(* Logix 5000 AddOnInstructionDefinition export EGU_EGK_Cyclic_Communication_1_0_3; software revision 35.00 *)

ADD_ON_INSTRUCTION EGU_EGK_Cyclic_Communication_1_0_3   (* revision 1.0 3, ExecutePrescan, ExecuteEnableInFalse *)
// Release 5.3.xxx
// ussed for EG Tested with:   V29.00.01 (CPR 9 SR 8.1) Built on: 08/11/16 01:38:38
//                 Schunk FW release 5.x
//  Engineering:   Studio 5000 V29.00.01 (CPR 9 SR 8.1) Built on: 08/11/16 01:38:38U / EGK Gripper
// Revision note:
// Change for Firmware 5.3
VAR_INPUT
   b_in_RELEASE_FUNCTION_BLOCK : BOOL; {access Read Only, visible}
   b_in_00_FAST_STOP : BOOL; {access Read Only, visible}
   b_in_01_STOP : BOOL; {access Read Only, visible}
   b_in_02_ACKNOLEDGE : BOOL; {access Read Only, visible}
   b_in_03_PREPARE_FOR_SHUTDOWN : BOOL; {access Read Only, visible}
   b_in_04_SOFTRESET : BOOL; {access Read Only, visible}
   b_in_05_RELEASE_FOR_MANUAL_MOVEMENT : BOOL; {access Read Only, visible}
   b_in_06_REPEAT_COMMAND_TOGGLE : BOOL; {access Read Only, visible}
   b_in_07_GRIP_DIRECTION : BOOL; {access Read Only, visible}
   b_in_08_JOG_MODE_NEGATIVE : BOOL; {access Read Only, visible}
   b_in_09_JOG_MODE_POSITIVE : BOOL; {access Read Only, visible}
   b_in_11_RELEASE_WORKPIECE : BOOL; {access Read Only, visible}
   b_in_12_GRIP_WORKPIECE : BOOL; {access Read Only, visible}
   b_in_13_MOVE_TO_ABSOLUTE_POSITION : BOOL; {access Read Only, visible}
   b_in_14_MOVE_TO_RELATIVE_POSITION : BOOL; {access Read Only, visible}
   b_in_16_GRIP_WORKPIECE_AT_EXPECTED_POS : BOOL; {access Read Only, visible}
   b_in_30_BRAKE_TEST : BOOL; {access Read Only, visible}
   b_in_31_ACTIVATE_GRIP_FORCE_AND_POS_MA : BOOL; {access Read Only, visible}
   di_in_POSITION : DINT; {access Read Only, visible}
   di_in_VELOCITY : DINT; {access Read Only, visible}
   di_in_GRIPPING_FORCE : DINT; {access Read Only, visible}
END_VAR
VAR_OUTPUT
   b_out_00_READY_FOR_OPERATION : BOOL; {visible}
   b_out_01_CONTOL_AUTHORITY_FIELDBUS : BOOL; {visible}
   b_out_02_READY_FOR_SHUTDOWN : BOOL; {visible}
   b_out_03_NOT_FEASIBLE : BOOL; {visible}
   b_out_04_COMMAND_SUCCESSFULLY_PROCESSED : BOOL; {visible}
   b_out_05_COMMAND_RECEIVED_TOGGLE : BOOL; {visible}
   b_out_06_WARNING : BOOL; {visible}
   b_out_07_ERROR : BOOL; {visible}
   b_out_08_RELEASED_FOR_MANUAL_MOVEMENT : BOOL; {visible}
   b_out_09_SOFTWARE_LIMIT_REACHED : BOOL; {visible}
   b_out_11_NO_WORKPIECE_DETECTED : BOOL; {visible}
   b_out_12_WORKPIECE_GRIPPED : BOOL; {visible}
   b_out_13_POSITION_REACHED : BOOL; {visible}
   b_out_14_WORKPIECE_PRE_GRIP_STARTED : BOOL; {visible}
   b_out_16_WORKPIECE_LOST : BOOL; {visible}
   b_out_17_WRONG_WORKPIECE_DETECTED : BOOL; {visible}
   b_out_31_GRIP_FORCE_AND_POS_MAINTAINANC : BOOL; {visible}
END_VAR
VAR_INPUT
   di_out_ACTUAL_POSITION : DINT; {visible}
END_VAR
VAR_OUTPUT
   si_out_DIAGNOSIS_ERROR : SINT; {visible}
   si_out_DIAGNOSIS_WARNING : SINT; {visible}
   si_out_DIAGNOSIS_WARNING_CODE : SINT; {visible}
END_VAR
VAR_INPUT
   di_in_INPUT_DATA_GRIPPER_DW_0 : DINT; {access Read Only, required}
   di_in_INPUT_DATA_GRIPPER_DW_1 : DINT; {access Read Only, required}
   di_in_INPUT_DATA_GRIPPER_DW_3 : DINT; {access Read Only, required}
END_VAR
VAR_OUTPUT
   di_out_OUTPUT_DATA_Gripper_DW_0 : DINT; {required}
   di_out_OUTPUT_DATA_Gripper_DW_1 : DINT; {required}
   di_out_OUTPUT_DATA_Gripper_DW_2 : DINT; {required}
   di_out_OUTPUT_DATA_Gripper_DW_3 : DINT; {required}
END_VAR
VAR
   stat_Input : DINT[4]; {access None}
   stat_Output : DINT[4]; {access None}
END_VAR

ROUTINE EnableInFalse   (* structured text *)
   //////////////////////////////////////////////////////////////
   //   Copyright (c)  <Company Information>
   //--------------------------------------------------------------
   //   Routine: <Routine Name>
   //       Author: <Developer Name>
   //   Created: <Date>
   //--------------------------------------------------------------
   //   Description:
   //
   //   History:
   //
   /////////////////////////////////////////////////////////////
END_ROUTINE

ROUTINE Logic   (* structured text *)
   
   (*
   FUNCTION_BLOCK FB_SFP_EGU/EGK Allen Breadley
   TITLE = 'EGU_EGK_Cyclic_Communication'
   VERSION : '1.0.3'
   AUTHOR  : 'SCHUNK'
   NAME    : 'EGU_EGK_Cyclic_Communication'
   FAMILY  : 'SCHUNK'
   Used Products : EGU / EGK
   Projekt Nr.:
   =============================================================================
    Schunk GmbH&Co.KG
    (c)Copyright (2022) All Rights Reserved
   -----------------------------------------------------------------------------
    Library:       Schunk
    Tested with:   V35.00.00
                   Schunk FW release 5.x
    Engineering:   Studio 5000 V35.00.00
    Restrictions:  XXX(OB types, etc.)
    Requirements:  (hardware, technological package, memory needed, etc.)
    Functionality: The Funktion Block communicates Cyclic with the Gripper to read and wright Data
   
   *************************************************************************
   Historie
   ####################
   1.0.3
   - Compartible with FW 5.3 Protokol
   - order when deleting bits changed
   ####################
   1.0.2
   - Compartible with FW 5.2 Protokol
   - New Bit "Brake Test"
   - Changesd Bit Names not the Funktions behind
   ####################
   1.0.1
   Bugfix
   	di_out_OUTPUT_DATA_Gripper_DW_2 := di_in_VELOCITY;
   	di_out_OUTPUT_DATA_Gripper_DW_3 := di_in_GRIPPING_FORCE;
   ####################
   1.0.0
   Release Funktion Block
   TagType="Base" DataType="BOOL" Usage="Input" Radix="Binary" Required="false" Visible="true" ExternalAccess="Read Only"
   
   *************************************************************************)
   	(*English
   
       Statement section REGION
   
       *************************************************************************
       The function block is TO read AND transfer cyclic parameters that are changed FOR specific functions in the device
       can be used TO make The application process safer OR faster.
   
       Input parameters:
       ------------------
       b_in_RELEASE_FUNCTION_BLOCK				: Release FOR processing the block
   
       b_in_00_FAST_STOP						: immediate shutdown OF The process currently running in The gripper AND shutdown OF The motor phases
       b_in_01_STOP							: Pausing AND stopping the currently running process.
       b_in_02_ACKNOLEDGE						: Acknowledge fault
       b_in_03_PREPARE_FOR_SHUTDOWN			: Initiate the restoration OF data on The device in preparation FOR switching off OR rebooting
       b_in_04_SOFTRESET						: Warm start OF The device
       b_in_05_RELEASE_FOR_MANUAL_MOVEMENT		: The brake can be released FOR 5 seconds in the "ERROR_FAST_STOP" state
       b_in_06_REPEAT_COMMAND_TOGGLE			: The command that is still pending can, IF it is a repeatable command, be repeated without loss OF Time FOR each positive AND negative change OF this bit
       b_in_07_GRIP_DIRECTION					: determines The gripping direction. FALSE = external gripping (the workpiece is gripped from the outside) / True = internal gripping (the workpiece is gripped from the inside).
   
       b_in_08_JOG_MODE_NEGATIVE				: Simple movement OF The device in negative direction. Function also possible without "REFERENCE".
       b_in_09_JOG_MODE_POSITIVE				: Simple movement OF The device in The positive direction. Function also possible without "REFERENCE".
   
       b_in_11_RELEASE_WORKPIECE				: IF The status is "GRIPPED", the gripper is opened in the opposite direction AND the workpiece is released
       b_in_12_GRIP_WORKPIECE					: the gripper executes a movement that should lead TO gripping a workpiece. Internal speed parameters are used here
       b_in_13_MOVE_TO_ABSOLUTE_POSITION		: the gripper jaws are moved TO The position specified in The cyclic protocol at The specified speed.
       b_in_14_MOVE_TO_RELATIVE_POSITION		: the gripper jaws are moved TO The calculated position with The position specified in The cyclic protocol at The specified speed.
   
       b_in_16_GRIP_WORKPIECE_AT_EXPECTED_POSITION :  the gripper performs a gripping run on a specified workpiece. first a positioning run to the pre-position and then a gripping run to the workpiece.
       b_in_30_BRAKE_TEST						: the gripper activates the brake and energizes the motor
   	b_in_31_ACTIVATE_GRIP_FORCE_AND_POSITION_MAINTENANCE  :  sets the use of gripping force and position maintenance ( False = GPE is not used / True = GPE is activated)
   
       di_in_POSITION							: Entry of the absolute or relative position in µm
       di_in_VELOCITY							: Entry of the speed when positioning gripping mm/sec
       di_in_GRIPPING_FORCE					: Entry of the gripping force is entered in %. Here you can read in the manual which gripping modes should be used. The indication of the gripping force can then be selected accordingly.
   
       di_in_INPUT_DATA_GRIPPER_DW_0			: Input Data DoubleWord 0 of the Gripper
       di_in_INPUT_DATA_GRIPPER_DW_1			: Input Data DoubleWord 1 of the Gripper
       di_in_INPUT_DATA_GRIPPER_DW_2			: Input Data DoubleWord 2 of the Gripper
       di_in_INPUT_DATA_GRIPPER_DW_3			: Input Data DoubleWord 3 of the Gripper
   
       #################
   
       Output parameters:
       ------------------
   
       b_out_00_READY_FOR_OPERATION            : indicates that the gripper is ready FOR operation
       b_out_01_CONTOL_AUTHORITY_FIELDBUS      : indicates whether the fieldbus has control authority over the gripper
       b_out_02_READY_FOR_SHUTDOWN             : signals readiness FOR shutdown OR restart after the request "Prepare for shutdown"
       b_out_03_NOT_FEASIBLE                   : Indicates that the last issued command cannot be executed.
                                               Possible causes are:
                                               - a new command was sent although the command that is still active has NOT yet been processed.
                                               - 2 OR more control commands simultaneously active in the control word
                                               - Parameter data FOR position, speed OR force are outside the permissible limits.
   
       b_out_04_COMMAND_SUCCESSFULLY_PROCESSED : indicates that the last executable command was successfully processed.
       b_out_05_COMMAND_RECEIVED_TOGGLE        : indicates that a command was sent TO The gripper via The bus. the command does NOT have TO be processed OR started at the time it is displayed.
       b_out_06_WARNING                        : signals a warning in the gripper, e.g. temperature warning
       b_out_07_ERROR                          : signals a fault in the gripper, e.g. rapid stop
       b_out_08_RELEASD_FOR_MANUAL_MOVEMENT    : Signals that the brake is released IF a brake is installed in the gripper.
       b_out_09_SOFTWARELIMIT_REACHED          : indicates that the gripper has reached a software limit
   
       b_out_11_NO_WORKPIECE_DETECTED          : indicates that no workpiece was detected
       b_out_12_WORKPIECE_GRIPPED              : signals that a workpiece has been gripped
       b_out_13_POSITION_REACHED               : signals that the relative OR absolute position has been approached
       b_out_14_WORKPIECE_PRE_GRIPPED_STARTED  : indicates that the gripper has started the pre-gripping function
       b_out_16_WORKPIECE_LOST                 : signals that the gripped workpiece was lost
       b_out_17_WRONG_WORKPIECE_DETECTED       : signals that a wrong workpiece was detected
       b_out_31_GRIP_FORCE_AND_POSITION_MAINTAINANCE_ACTIVATED : signals that GPE is active
   
       di_out_ACTUAL_POSITION                  : the current position OF The gripper is returned here
       i_out_DIAGNOSE_WARNUNG                  : Output of the gripper's warning code
       i_out_DIAGNOSE_ERROR                    : Output of the error code of the gripper
   
       di_out_OUTPUT_DATA_Gripper_DW_0			: Output Data DoubleWord 0 of the Gripper
       di_out_OUTPUT_DATA_Gripper_DW_1			: Output Data DoubleWord 1 of the Gripper
       di_out_OUTPUT_DATA_Gripper_DW_2			: Output Data DoubleWord 2 of the Gripper
       di_out_OUTPUT_DATA_Gripper_DW_3			: Output Data DoubleWord 3 of the Gripper
   
       *************************************************************************)
   
   
   (*************************************************************************
       German
   
   	Der Baustein soll Zyklische Parameter einlesen und übertragen, welche für bestimmte Funktionen im Gerät geändert
       werden können um den Applikationsprozess sicherer oder schneller zu machen.
   
       Eingangsparameter:
       ------------------
   
       b_RELEASE_FUNCTION_BLOCK            : Freigabe zur Bearbeitung des Bausteins (True = Freigabe zur Bearbeitung)
   
       b_00_FAST_STOP                      : sofortiges Abschalten des aktuell im Greifer laufenden Prozesses und abschalten der Motorphasen
       b_01_STOP                           : Anhalten und Stoppen des Aktuell laufenden Prozesses.
       b_02_ACKNOLEDGE                     : Störung Quittieren
       b_03_PREPARE_FOR_SHUTDOWN           : Anstoßen der Rückspeicherung von Daten auf dem Grät un Vorbereitung zum Ausschalten oder Reboot
       b_04_SOFTRESET                      : Warmstart des Gerätes
       b_05_RELEASE_FOR_MANUAL_MOVEMENT    : Lösen der Bremse für 5 Sekunden im Zustand "ERROR_FAST_STOP" möglich
       b_06_REPEAT_COMMAND_TOGGLE          : Das Noch anstehende Kommando kann, sofern es ein wiederholbares Kommando ist, ohne zeitverlust bei jedem positiven und negativen wechsel dieses Bits wiederholt werden
       b_07_GRIP_DIRECTION                 : legt die Greifrichtung fest. FALSE = Ausengreifen (Das Werkstück wird von ausen gegriffen) / True = Innengreifen (Das Werkstück wird von innen gegriffen).
   
       b_08_JOG_MODE_NEGATIVE              : einfaches Verfahren des Gerätes in negative Richtung. Funktion auch ohne Referenz möglich.
       b_09_JOG_MODE_POSITIVE              : einfaches Verfahren des Gerätes in positive Richtung. Funktion auch ohne Referenz möglich.
   
       b_11_RELEASE_WORKPIECE              : Bei Status "GRIPPED" wird der Greifer in die entgegegesetzte Richtung geöffnet und das Werkstück freigegeben
       b_12_GRIP_WORKPIECE                 : der Greifer führt eine Bewegung aus, welche zum greifen eines Werkstückes führen soll. Hierbei werden interne Geschwindigkeitsparameter genommen
       b_13_MOVE_TO_ABSOLUTE_POSITION      : Die Greiferbacken werden auf die im Zyklischen Protokoll vorgegebene Position mit der vorgegebenen Geschwindigkeit gefahren.
       b_14_MOVE_TO_RELATIVE_POSITION      : Die Greiferbacken werden auf die errechnete Position mit der im Zyklischen Protokoll vorgegebene Position mit der vorgegebenen Geschwindigkeit gefahren.
   
       b_16_GRIP_WORKPIECE_AT_EXPECTED_POSITION            : Der Greifer führt eine Greiffahrt auf ein vorgegebenes Werkstück aus. Hierbei wird zuerst eine Positionsfahrt auf die Vorposition um dann mit einer Greiffahrt auf das Werkstück zu fahren.
       b_in_30_BRAKE_TEST						: der Greifer aktiviert die Bremse und bestromt den Motor
   	b_31_ACTIVATE_GRIP_FORCE_AND_POSITION_MAINTENANCE   : legt die Verwendung der Greifkaft und Positionserhaltung fest ( False = GPE wird nicht verwendet / True = GPE wird aktiviert)
   
       di_POSITION                         : Eintrag der Absoluten oder Relativen Possition in µm
       di_VELOCITY                         : Eintrag der Geschwindigkeit beim Possitioniern Greifen mm/Sec
       di_GRIPPING_FORCE                   : Eintrag der Greifkraft wird in % eingetragen. Hier ist im Handbuch nachzulesen welcher Greifmodi verwendet werden soll. Entsprechend kann dann die angabe der Greifkraft gewählt werden.
   
       di_in_INPUT_DATA_GRIPPER_DW_0		:	Eingangsdaten Doppelwort 0 des Greifers
       di_in_INPUT_DATA_GRIPPER_DW_1		:	Eingangsdaten Doppelwort 1 des Greifers
       di_in_INPUT_DATA_GRIPPER_DW_2		:	Eingangsdaten Doppelwort 2 des Greifers
       di_in_INPUT_DATA_GRIPPER_DW_3		:   Eingangsdaten Doppelwort 3 des Greifers
   
       ##################
   
   
       Ausgangsparameter:
       ------------------
   
       b_out_00_READY_FOR_OPPERATION           : zeigt die Betriebsbereitschaft des Greifers an
       b_out_01_CONTOL_AUTHORITY_FIELDBUS      : zeigt an, ob der Feldbus die Steuerhoheit über den Greifer hat
       b_out_02_READY_FOR_SHUTDOWN             : signalisiert die Bereitschaft zum Abschalten bzw Neustarten nach der Anforderung "Prepare for shutdown"
       b_out_03_NOT_FEASIBLE                   : Zeigt an, das der zuletzt abgesetzte Befehl nicht ausgeführt werden kann.
                                               Mögliche Ursachen sind:
                                               - ein neuer Befehl wurde abgesetzt, obwohl der noch aktive Befehl noch nicht abgearbeitet wurde.
                                               - 2 oder mehr Steuerbefehle gleichzeitig aktiv im Steuerwort
                                               - Parameterdaten von Position, Geschwindigkeit oder Kraft liegen auserhalb der Zulässigen grenzen.
   
       b_out_04_COMMAND_SUCCESSFULLY_PROCESSED : zeigt das erfolgreiche Abarbeiten des letzten ausführbaren Befehls an.
       b_out_05_COMMAND_RECEIVED_TOGGLE        : Zeigt an, das ein Befehl über den Bus an den Greufer gesendet wurde. Zum Zeitpunkt der Anzeige muß der Befehl noch nicht abgearbeitet oder gestartet sein.
       b_out_06_WARNING                        : signalisiert eine Warnung im Greifer, z.B. Temperaturwarnung
       b_out_07_ERROR                          : signalisiert eine Störung im Greifer, z.B. Schnellstop
       b_out_08_RELEASD_FOR_MANUAL_MOVEMENT    : Signalisiert, dass die Bremse geöffnet ist, sofern eine Bremse im Greifer verbaut ist.
       b_out_09_SOFTWARELIMIT_REACHED          : signalisiert, das der Greifer eine Softwarelimit angefahren hat
       b_out_10_REFERENCED                     : signalisiert, das der Greifer referenziert ist
       b_out_11_NO_WORKPIECE_DETECTED          : signalisiert, dass kein Werkstück erkannt wurde
       b_out_12_WORKPIECE_GRIPPED              : signalisiert, dass ein Werkstück gegriffen wurde
       b_out_13_POSITION_REACHED               : signalisiert, dass die relative oder absolute Possition angefahren wurde
       b_out_14_WORKPIECE_PRE_GRIPPED_STARTED  : signalisiert, dass der Greifer die Pre Gripping Funktion angestoßen hat
       b_out_16_WORKPIECE_LOST                 : signalisiert, dass das gegriffene Werkstück verloren ging
       b_out_17_WRONG_WORKPIECE_DETECTED       : signalisiert, das ein falsches Werkstück erkannt wurde
       b_out_31_GRIP_FORCE_AND_POSITION_MAINTAINANCE_ACTIVATED :   Signalisiert, dass GPE aktiev ist
   
       di_out_ACTUAL_POSITION                  : hier wird die aktuelle Possition des Greifers zurückgegeben
       i_out_DIAGNOSE_WARNUNG                  : Ausgabe des Warnungscodes des Greifers
       i_out_DIAGNOSE_ERROR                    : Ausgabe des Störungscodes des Greifers
   
       di_out_OUTPUT_DATA_Gripper_DW_0		: Output Data DoubleWord 0 of the Gripper
       di_out_OUTPUT_DATA_Gripper_DW_1		: Output Data DoubleWord 1 of the Gripper
       di_out_OUTPUT_DATA_Gripper_DW_2		: Output Data DoubleWord 2 of the Gripper
       di_out_OUTPUT_DATA_Gripper_DW_3		: Output Data DoubleWord 3 of the Gripper
   *************************************************************************)
   
   
   
   
       // Enter the input data in the instance DB and assign them to the status displays
       // Eingangsdaten in den Instanz DB eintragen und den Statusanzeigen zuweisen
   
   	b_out_00_READY_FOR_OPERATION 			:= di_in_INPUT_DATA_GRIPPER_DW_0.0;
   	b_out_01_CONTOL_AUTHORITY_FIELDBUS 		:= di_in_INPUT_DATA_GRIPPER_DW_0.1;
   	b_out_02_READY_FOR_SHUTDOWN 			:= di_in_INPUT_DATA_GRIPPER_DW_0.2;
   	b_out_03_NOT_FEASIBLE 					:= di_in_INPUT_DATA_GRIPPER_DW_0.3;
   	b_out_04_COMMAND_SUCCESSFULLY_PROCESSED := di_in_INPUT_DATA_GRIPPER_DW_0.4;
   	b_out_05_COMMAND_RECEIVED_TOGGLE 		:= di_in_INPUT_DATA_GRIPPER_DW_0.5;
   	b_out_06_WARNING 						:= di_in_INPUT_DATA_GRIPPER_DW_0.6;
   	b_out_07_ERROR 							:= di_in_INPUT_DATA_GRIPPER_DW_0.7;
   	b_out_08_RELEASED_FOR_MANUAL_MOVEMENT 	:= di_in_INPUT_DATA_GRIPPER_DW_0.8;
   	b_out_09_SOFTWARE_LIMIT_REACHED 		:= di_in_INPUT_DATA_GRIPPER_DW_0.9;
   	b_out_11_NO_WORKPIECE_DETECTED 			:= di_in_INPUT_DATA_GRIPPER_DW_0.11;
   	b_out_12_WORKPIECE_GRIPPED 				:= di_in_INPUT_DATA_GRIPPER_DW_0.12;
   	b_out_13_POSITION_REACHED 				:= di_in_INPUT_DATA_GRIPPER_DW_0.13;
   	b_out_14_WORKPIECE_PRE_GRIP_STARTED 	:= di_in_INPUT_DATA_GRIPPER_DW_0.14;
   	b_out_16_WORKPIECE_LOST 				:= di_in_INPUT_DATA_GRIPPER_DW_0.16;
   	b_out_17_WRONG_WORKPIECE_DETECTED 		:= di_in_INPUT_DATA_GRIPPER_DW_0.17;
   	b_out_31_GRIP_FORCE_AND_POS_MAINTAINANC := di_in_INPUT_DATA_GRIPPER_DW_0.31;
   
   
   	di_out_ACTUAL_POSITION 			:= di_in_INPUT_DATA_GRIPPER_DW_1;
   
   	si_out_DIAGNOSIS_ERROR.0 			:= di_in_INPUT_DATA_GRIPPER_DW_3.0;
   	si_out_DIAGNOSIS_ERROR.1 			:= di_in_INPUT_DATA_GRIPPER_DW_3.1;
   	si_out_DIAGNOSIS_ERROR.2 			:= di_in_INPUT_DATA_GRIPPER_DW_3.2;
   	si_out_DIAGNOSIS_ERROR.3 			:= di_in_INPUT_DATA_GRIPPER_DW_3.3;
   	si_out_DIAGNOSIS_ERROR.4 			:= di_in_INPUT_DATA_GRIPPER_DW_3.4;
   	si_out_DIAGNOSIS_ERROR.5 			:= di_in_INPUT_DATA_GRIPPER_DW_3.5;
   	si_out_DIAGNOSIS_ERROR.6 			:= di_in_INPUT_DATA_GRIPPER_DW_3.6;
   	si_out_DIAGNOSIS_ERROR.7 			:= di_in_INPUT_DATA_GRIPPER_DW_3.7;
   
   	si_out_DIAGNOSIS_WARNING.0 			:= di_in_INPUT_DATA_GRIPPER_DW_3.16;
   	si_out_DIAGNOSIS_WARNING.1 			:= di_in_INPUT_DATA_GRIPPER_DW_3.17;
   	si_out_DIAGNOSIS_WARNING.2 			:= di_in_INPUT_DATA_GRIPPER_DW_3.18;
   	si_out_DIAGNOSIS_WARNING.3			:= di_in_INPUT_DATA_GRIPPER_DW_3.19;
   	si_out_DIAGNOSIS_WARNING.4 			:= di_in_INPUT_DATA_GRIPPER_DW_3.20;
   	si_out_DIAGNOSIS_WARNING.5 			:= di_in_INPUT_DATA_GRIPPER_DW_3.21;
   	si_out_DIAGNOSIS_WARNING.6 			:= di_in_INPUT_DATA_GRIPPER_DW_3.22;
   	si_out_DIAGNOSIS_WARNING.7 			:= di_in_INPUT_DATA_GRIPPER_DW_3.23;
   
   	si_out_DIAGNOSIS_WARNING_CODE.0 	:= di_in_INPUT_DATA_GRIPPER_DW_3.24;
   	si_out_DIAGNOSIS_WARNING_CODE.1 	:= di_in_INPUT_DATA_GRIPPER_DW_3.25;
   	si_out_DIAGNOSIS_WARNING_CODE.2 	:= di_in_INPUT_DATA_GRIPPER_DW_3.26;
   	si_out_DIAGNOSIS_WARNING_CODE.3 	:= di_in_INPUT_DATA_GRIPPER_DW_3.27;
   	si_out_DIAGNOSIS_WARNING_CODE.4 	:= di_in_INPUT_DATA_GRIPPER_DW_3.28;
   	si_out_DIAGNOSIS_WARNING_CODE.5 	:= di_in_INPUT_DATA_GRIPPER_DW_3.29;
   	si_out_DIAGNOSIS_WARNING_CODE.6 	:= di_in_INPUT_DATA_GRIPPER_DW_3.30;
   	si_out_DIAGNOSIS_WARNING_CODE.7 	:= di_in_INPUT_DATA_GRIPPER_DW_3.31;
   
       // Allocation of output data for the periphery
       // Zuweisung der Ausgangsdaten für die Peripher
   
   
   
   	di_out_OUTPUT_DATA_Gripper_DW_0.0 := b_in_00_FAST_STOP;
   	di_out_OUTPUT_DATA_Gripper_DW_0.1 := b_in_01_STOP;
   	di_out_OUTPUT_DATA_Gripper_DW_0.2 := b_in_02_ACKNOLEDGE;
   	di_out_OUTPUT_DATA_Gripper_DW_0.3 := b_in_03_PREPARE_FOR_SHUTDOWN;
   	di_out_OUTPUT_DATA_Gripper_DW_0.4 := b_in_04_SOFTRESET;
   	di_out_OUTPUT_DATA_Gripper_DW_0.5 := b_in_05_RELEASE_FOR_MANUAL_MOVEMENT;
   	di_out_OUTPUT_DATA_Gripper_DW_0.6 := b_in_06_REPEAT_COMMAND_TOGGLE;
   	di_out_OUTPUT_DATA_Gripper_DW_0.7 := b_in_07_GRIP_DIRECTION;
   	di_out_OUTPUT_DATA_Gripper_DW_0.8 := b_in_08_JOG_MODE_NEGATIVE;
   	di_out_OUTPUT_DATA_Gripper_DW_0.9 := b_in_09_JOG_MODE_POSITIVE;
   	di_out_OUTPUT_DATA_Gripper_DW_0.10 := 0;
   	di_out_OUTPUT_DATA_Gripper_DW_0.11 := b_in_11_RELEASE_WORKPIECE;
   	di_out_OUTPUT_DATA_Gripper_DW_0.12 := b_in_12_GRIP_WORKPIECE;
   	di_out_OUTPUT_DATA_Gripper_DW_0.13 := b_in_13_MOVE_TO_ABSOLUTE_POSITION;
   	di_out_OUTPUT_DATA_Gripper_DW_0.14 := b_in_14_MOVE_TO_RELATIVE_POSITION;
   	di_out_OUTPUT_DATA_Gripper_DW_0.15 := 0;
   	di_out_OUTPUT_DATA_Gripper_DW_0.16 := b_in_16_GRIP_WORKPIECE_AT_EXPECTED_POS;
   	di_out_OUTPUT_DATA_Gripper_DW_0.17 := 0;
   	di_out_OUTPUT_DATA_Gripper_DW_0.18 := 0;
   	di_out_OUTPUT_DATA_Gripper_DW_0.19 := 0;
   	di_out_OUTPUT_DATA_Gripper_DW_0.20 := 0;
   	di_out_OUTPUT_DATA_Gripper_DW_0.21 := 0;
   	di_out_OUTPUT_DATA_Gripper_DW_0.22 := 0;
   	di_out_OUTPUT_DATA_Gripper_DW_0.23 := 0;
   	di_out_OUTPUT_DATA_Gripper_DW_0.24 := 0;
   	di_out_OUTPUT_DATA_Gripper_DW_0.25 := 0;
   	di_out_OUTPUT_DATA_Gripper_DW_0.26 := 0;
   	di_out_OUTPUT_DATA_Gripper_DW_0.27 := 0;
   	di_out_OUTPUT_DATA_Gripper_DW_0.28 := 0;
   	di_out_OUTPUT_DATA_Gripper_DW_0.29 := 0;
   	di_out_OUTPUT_DATA_Gripper_DW_0.30 := b_in_30_BRAKE_TEST;
   	di_out_OUTPUT_DATA_Gripper_DW_0.31 := b_in_31_ACTIVATE_GRIP_FORCE_AND_POS_MA;
   
   
   	di_out_OUTPUT_DATA_Gripper_DW_1 := di_in_POSITION;
   	di_out_OUTPUT_DATA_Gripper_DW_2 := di_in_VELOCITY;
   	di_out_OUTPUT_DATA_Gripper_DW_3 := di_in_GRIPPING_FORCE;
   
     IF NOT b_in_RELEASE_FUNCTION_BLOCK
   
       THEN
   
   		stat_Output[0].0 := 0;
   		stat_Output[0].1 := 0;
   		stat_Output[0].2 := 0;
   		stat_Output[0].3 := 0;
   		stat_Output[0].4 := 0;
   		stat_Output[0].5 := 0;
   		//stat_Output[0].6 := 0;
   		//stat_Output[0].7 := 0;
   		stat_Output[0].8 := 0;
   		stat_Output[0].9 := 0;
   		stat_Output[0].10 := 0;
   		stat_Output[0].11 := 0;
   		stat_Output[0].12 := 0;
   		stat_Output[0].13 := 0;
   		stat_Output[0].14 := 0;
   		stat_Output[0].15 := 0;
   		stat_Output[0].16 := 0;
   		stat_Output[0].17 := 0;
   		stat_Output[0].18 := 0;
   		stat_Output[0].19 := 0;
   		stat_Output[0].20 := 0;
   		stat_Output[0].21 := 0;
   		stat_Output[0].22 := 0;
   		stat_Output[0].23 := 0;
   		stat_Output[0].24 := 0;
   		stat_Output[0].25 := 0;
   		stat_Output[0].26 := 0;
   		stat_Output[0].27 := 0;
   		stat_Output[0].28 := 0;
   		stat_Output[0].29 := 0;
   		stat_Output[0].30 := 0;
   		stat_Output[0].31 := 0;
   
   		stat_Output[1] := 0;		//Position
   		stat_Output[2] := 0;		//Velocity
   		stat_Output[3] := 0;		//Gripping Force
   
       END_IF;
END_ROUTINE

ROUTINE Postscan   (* structured text *)
   //////////////////////////////////////////////////////////////
   //   Copyright (c)  <Company Information>
   //--------------------------------------------------------------
   //   Routine: <Routine Name>
   //       Author: <Developer Name>
   //   Created: <Date>
   //--------------------------------------------------------------
   //   Description:
   //
   //   History:
   //
   /////////////////////////////////////////////////////////////
END_ROUTINE

ROUTINE Prescan   (* structured text *)
   //////////////////////////////////////////////////////////////
   //   Copyright (c)  <Company Information>
   //--------------------------------------------------------------
   //   Routine: <Routine Name>
   //       Author: <Developer Name>
   //   Created: <Date>
   //--------------------------------------------------------------
   //   Description:
   //
   //   History:
   //
   /////////////////////////////////////////////////////////////
END_ROUTINE
END_ADD_ON_INSTRUCTION
